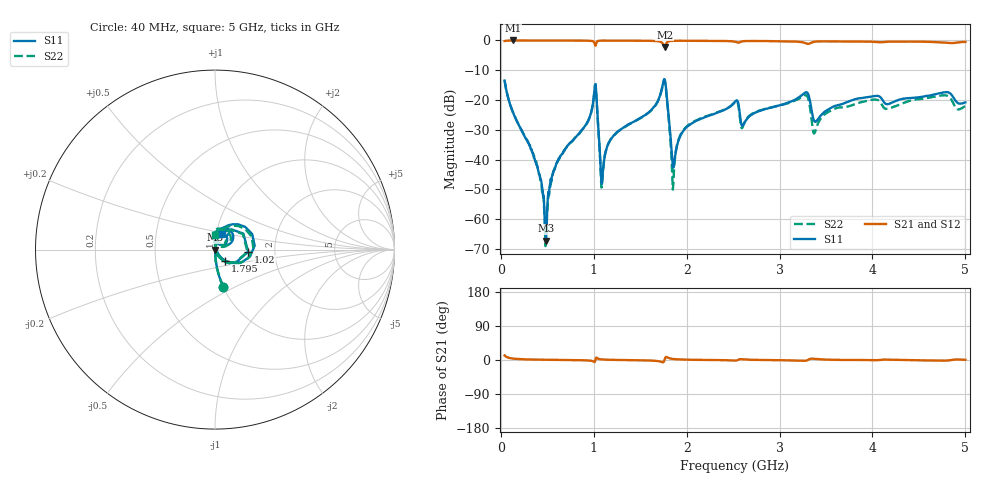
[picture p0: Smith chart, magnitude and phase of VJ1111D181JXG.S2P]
! VJ1111D181JXG
! DATE 02/15/2022  13:17
! CAPACITORS MOUNTED IN SERIES ON 25 MIL THICK MICROSTRIP SUBSTRATE
# GHz  S  MA  R  50.00
!  FREQ  S11M  S11A  S21M  S21A  S12M  S12A  S22M  S22A
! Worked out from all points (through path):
!   801 points, 40 MHz to 5 GHz, reference 50 ohm
!   highest |S21| = 0.00 dB at 126.8 MHz (marker M1); lowest = -2.2 dB at 1.764 GHz (marker M2)
!   lowest |S11| = -67.2 dB at 486.4 MHz (marker M3), VSWR 1.00, Z = 50 - j0.00302 ohm
!   |S11| at or under -10 dB: start of sweep to end of sweep
!   |S22| runs from -69.0 to -13.3 dB; largest |S21 - S12| = 0.0099
!   S11 on the Smith chart (normalised r, x): 40 MHz: 1.00, -0.43; 1.02 GHz: 1.45, -0.03; 1.795 GHz: 1.11, -0.14; 5 GHz: 1.05, +0.18
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0.04  0.2118 -77.2  0.9773 12.1  0.9777 12.3  0.2143 -77.7
0.1268  0.06345 -86.6  1 4.0  0.9978 3.9  0.0655 -84.8
0.3686  0.009455 -85.8  0.9967 1.1  1.001 1.0  0.0106 -86.7
0.4864  0.0004364 -4.0  0.9972 0.7  1 0.8  0.0007302 56.8
0.5918  0.008068 86.0  0.9964 0.3  1.001 0.5  0.008163 82.8
0.8708  0.03136 84.9  0.9943 -0.5  0.9977 -0.5  0.03098 86.1
1.0196  0.1853 -3.6  0.8156 2.6  0.8169 2.6  0.1813 -3.9
1.0692  0.0103 -54.5  0.9914 2.0  0.9941 2.0  0.009424 -56.2
1.094  0.00535 54.7  0.9939 1.3  0.9963 1.3  0.004988 62.9
1.1994  0.02352 85.3  0.9938 0.4  0.9978 0.4  0.02359 87.5
1.6954  0.1011 75.9  0.9684 -3.2  0.9726 -3.3  0.0994 74.6
1.7636  0.222 5.7  0.7756 2.2  0.7791 2.1  0.2138 2.5
1.7946  0.08191 -47.9  0.9468 6.5  0.9514 6.4  0.07653 -53.3
1.8566  0.007331 19.9  0.988 2.7  0.9915 2.5  0.004016 56.0
1.9868  0.03379 86.1  0.989 1.0  0.9942 0.9  0.03421 91.1
2.52  0.09389 68.8  0.9527 -1.5  0.9581 -1.6  0.09195 71.0
2.6068  0.03791 65.5  0.9712 1.8  0.9759 1.5  0.03673 76.7
3.2764  0.134 57.3  0.9059 -2.0  0.9102 -2.2  0.1204 57.3
3.3508  0.06009 23.5  0.9293 3.6  0.9336 3.4  0.03882 23.1
3.977  0.1134 74.0  0.9539 -0.4  0.9584 -0.5  0.09982 88.8
4.1754  0.08604 70.8  0.955 0.7  0.9611 0.6  0.07231 87.6
5  0.09142 69.7  0.9459 0.5  0.9511 0.3  0.07948 89.2
